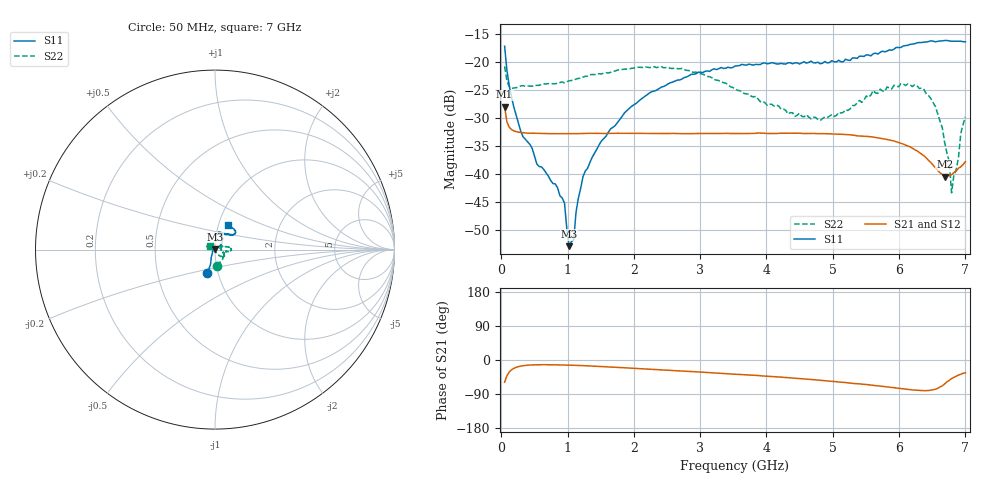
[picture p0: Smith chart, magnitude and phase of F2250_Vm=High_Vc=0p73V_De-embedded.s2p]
! Integrated Device Technology
! Corporate Headquarters
! 6024 Silver Creek Valley Road
! San Jose, CA 95138  USA
! Phone:  1-408-284-8200
! Toll Free:  1-800-223-1366
! Webpage:  http://www.idt.com/
! Timing and RF Division
! 515 Groton Road, Suite 102
! Westford, MA 01886-6024
! Device:  F2250
! Description: Voltage Variable RF Attenuator
! Frequency:  50.0 -  6000.00 MHz
! Package:  3x3 mm Thin QFN Plastic Package: 16 pin
! Ports:  2 RF, 3 DC
!  Pin  1  = GND
!  Pin  2  = NC
!  Pin  3  = RF1  = Port 1
!  Pin  4  = NC
!  Pin  5  = GND
!  Pin  6  = GND
!  Pin  7  = GND
!  Pin  8  = GND
!  Pin  9  = NC
!  Pin 10  = RF2  = Port 2
!  Pin 11  = NC
!  Pin 12  = GND
!  Pin 13  = GND
!  Pin 14  = VCNTRL
!  Pin 15  = VDD
!  Pin 16  = VMODE
! Vcntrl:  0.730 Volts
! Vmode:  +3.300 Volts
! Vdd:  +3.30  Volts
! Current:  1.293 mA
! Data:  The device was measured on a the F2250 evaluation board which has
!  individual transmission lines to the RF pins.  Data was collected
!  using a calibrated network analyzer.  The evaluation board was
!  de-embedded using a TRL calibration technique.
!  The reference plane is the edge of the package pin.
! Misc:  SN 10
!  Action Tracker AT0258
! Date Measured:  2014-11-26
! Date:  2015-10-15  MJV
! Note:
!  Integrated Device Technology supplies this data as a sample of measured
!  data at the package pin for this product.  Your particular data for this
!  product may vary.
!  Data was taken at 25 degrees C.
!  Integrated Device Technology reserves the right to change this data at anytime.
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# GHz S dB R 50
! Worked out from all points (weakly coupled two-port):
!   201 points, 50 MHz to 7 GHz, reference 50 ohm
!   highest |S21| = -27.98 dB at 50 MHz (marker M1); lowest = -40.5 dB at 6.687 GHz (marker M2)
!   lowest |S11| = -53.0 dB at 1.023 GHz (marker M3), VSWR 1.00, Z = 49.8 + j0.158 ohm
!   |S11| at or under -10 dB: start of sweep to end of sweep
!   |S22| runs from -43.4 to -20.8 dB; largest |S21 - S12| = 6.7e-05
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0.05  -17.15 -108.0  -27.98 -58.8  -27.97 -58.8  -20.76 -83.5
0.1195  -24.20 -111.2  -31.66 -31.7  -31.66 -31.7  -24.37 -35.7
0.29325  -32.37 -125.8  -32.60 -16.1  -32.61 -16.1  -24.26 -15.5
0.9535  -45.24 172.2  -32.82 -13.2  -32.83 -13.3  -23.71 -8.6
1.023  -52.96 135.4  -32.80 -13.6  -32.82 -13.6  -23.35 -8.2
1.0925  -51.83 75.5  -32.81 -14.0  -32.82 -13.9  -23.24 -7.9
1.12725  -46.90 52.5  -32.80 -14.1  -32.80 -14.2  -23.03 -8.4
1.2315  -40.55 36.8  -32.79 -14.9  -32.79 -14.9  -22.67 -9.2
1.6485  -31.94 39.7  -32.77 -18.5  -32.76 -18.5  -21.84 -6.1
2.37825  -24.75 46.0  -32.79 -25.6  -32.79 -25.7  -20.86 0.1
3.525  -20.69 71.4  -32.79 -37.4  -32.80 -37.4  -24.76 16.0
4.7065  -20.11 71.8  -32.77 -51.9  -32.77 -51.9  -29.86 17.2
5.01925  -19.94 63.1  -32.88 -56.8  -32.86 -56.8  -29.73 5.9
5.85325  -17.82 40.3  -33.94 -71.7  -33.94 -71.9  -24.60 -28.1
6.3745  -16.42 40.8  -36.77 -80.9  -36.78 -80.9  -24.89 -43.3
6.54825  -16.36 44.5  -38.91 -77.1  -38.93 -77.1  -27.97 -55.4
6.68725  -16.13 47.6  -40.50 -63.1  -40.49 -63.1  -34.43 -67.3
6.75675  -16.21 50.4  -40.32 -53.8  -40.33 -53.7  -37.81 -87.2
6.7915  -16.27 51.2  -40.18 -48.7  -40.15 -48.7  -43.40 -116.2
6.89575  -16.24 56.3  -39.00 -39.7  -39.00 -39.7  -37.11 158.4
6.9305  -16.26 58.6  -38.75 -37.7  -38.71 -37.8  -32.77 155.1
7  -16.36 62.2  -37.84 -33.8  -37.82 -33.6  -29.78 147.5
